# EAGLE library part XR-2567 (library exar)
Dual monolithic REGULATOR
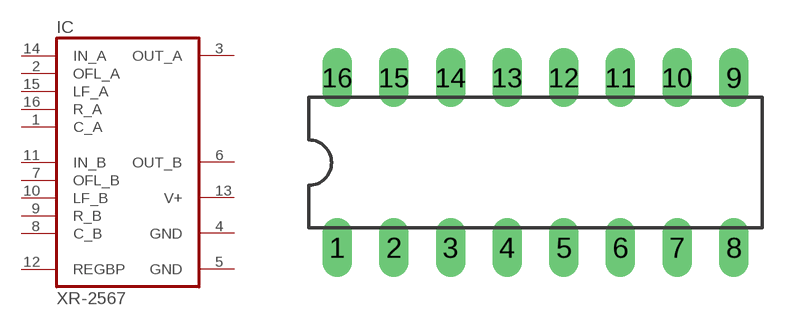
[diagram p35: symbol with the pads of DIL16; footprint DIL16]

Designator prefix IC

## XR-2567 (OC_FARNELL: unknown; OC_NEWARK: unknown)  [DIL16]
1  C_A  in
2  OFL_A  in
3  OUT_A  out
4  GND  pwr
5  GND  pwr
6  OUT_B  out
7  OFL_B  in
8  C_B  in
9  R_B  in
10  LF_B  in
11  IN_B  in
12  REGBP  in
13  V+  pwr
14  IN_A  in
15  LF_A  in
16  R_A  in

## Footprint DIL16 (pad centres in mm)
Dual In Line Package
drill 0.813 long: 1 -8.89,-3.81; 2 -6.35,-3.81; 3 -3.81,-3.81; 4 -1.27,-3.81; 5 1.27,-3.81; 6 3.81,-3.81; 7 6.35,-3.81; 8 8.89,-3.81; 9 8.89,3.81; 10 6.35,3.81; 11 3.81,3.81; 12 1.27,3.81; 13 -1.27,3.81; 14 -3.81,3.81; 15 -6.35,3.81; 16 -8.89,3.81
